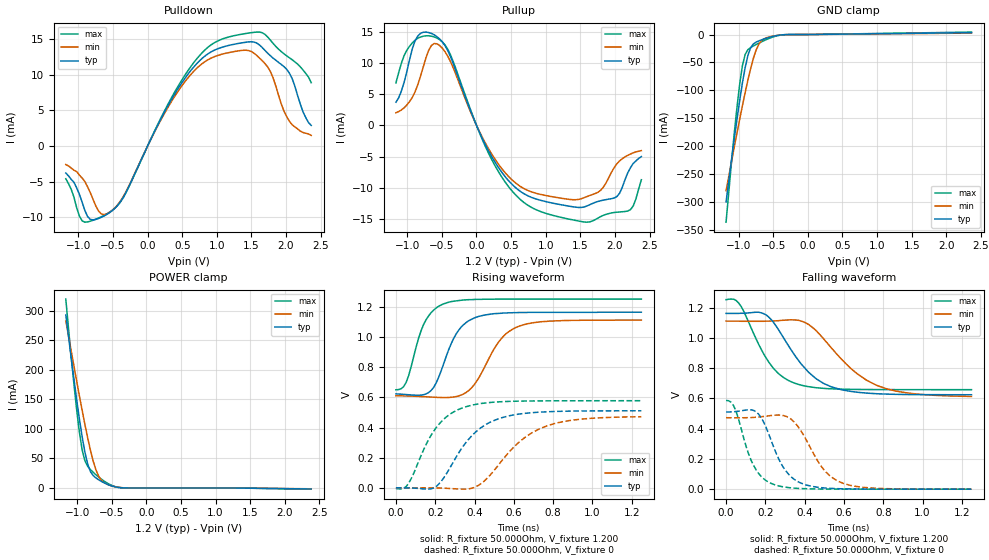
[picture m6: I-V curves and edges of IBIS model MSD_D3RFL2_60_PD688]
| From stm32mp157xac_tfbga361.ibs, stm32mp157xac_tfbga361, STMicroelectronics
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[Model] MSD_D3RFL2_60_PD688
Model_type   I/O
C_comp 2.461pF   2.375pF   2.586pF
Vinh = 820.000mV
Vinl = 380.000mV
Vmeas = 600.000mV
Vref = 600.000mV
[Model Spec]
Vinh   820.000mV   790.000mV   870.000mV
Vinl   380.000mV   350.000mV   430.000mV
Vmeas   600.000mV   570.000mV   650.000mV
Vref   600.000mV   570.000mV   650.000mV
[Temperature Range]   25.000   125.000   -40.000
[Voltage Range]   1.200V   1.140V   1.300V
[GND Clamp Reference]   0.00V   0.00V   0.00V
[Pulldown Reference]   0.00V   0.00V   0.00V
[POWER Clamp Reference]   1.200V   1.140V   1.300V
[Pullup Reference]   1.200V   1.140V   1.300V
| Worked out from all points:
|   slope of the pulldown table from 0 to 0.18 V, typ, clamps not added: 50.1 ohm
|   slope of the pullup table from 0 to 0.18 V, typ, clamps not added: 42.9 ohm
|   GND clamp passes 1 mA (typ) near -0.40 V on its own axis
|   POWER clamp passes 1 mA (typ) near -0.41 V on its own axis
|   rising waveform, R_fixture 50.000Ohm, V_fixture 1.200: 20-80 % time 109ps typ, 140ps min, 91.6ps max; typ from 0.623 V to 1.16 V
|   rising waveform, R_fixture 50.000Ohm, V_fixture 0: 20-80 % time 183ps typ, 224ps min, 153ps max; typ from 0.001 V to 0.511 V
|   falling waveform, R_fixture 50.000Ohm, V_fixture 1.200: 20-80 % time 190ps typ, 242ps min, 153ps max; typ from 1.16 V to 0.625 V
|   falling waveform, R_fixture 50.000Ohm, V_fixture 0: 20-80 % time 113ps typ, 138ps min, 96.4ps max; typ from 0.51 V to 0 V
[GND Clamp]
-1.182V   -299.6mA   -279.7mA   -335.9mA
-1.064V   -187.4mA   -201.8mA   -177.5mA
-984.9mV  -117.9mA   -151.6mA   -88.6mA
-945.5mV  -86.54mA   -127.3mA   -55.77mA
-906.1mV  -59.13mA   -104mA     -35.64mA
-866.7mV  -37.61mA   -81.71mA   -27.22mA
-827.3mV  -23.8mA    -61.15mA   -23.42mA
-748.5mV  -13.62mA   -28.14mA   -17.95mA
-709.1mV  -11.42mA   -17.52mA   -15.44mA
-630.3mV  -7.875mA   -7.542mA   -10.71mA
-472.7mV  -2.454mA   -2.156mA   -3.182mA
2.364V    3.327mA    2.556mA    4.357mA
[Power Clamp]
-1.164V   292.5mA    282.6mA    319.4mA
-1.085V   218.7mA    230.9mA    220.2mA
-1.006V   148.5mA    180.1mA    131.2mA
-966.7mV  115.9mA    155.2mA    93.42mA
-927.3mV  86.16mA    130.9mA    64.04mA
-887.9mV  60.43mA    107.4mA    45.92mA
-809.1mV  27.85mA    64.33mA    31.18mA
-730.3mV  17.06mA    31.16mA    22.45mA
-651.5mV  11.24mA    13.38mA    14.99mA
-533.3mV  4.769mA    4.703mA    6.239mA
-336.4mV  190.8uA    361uA      219.4uA
2.382V    -1.713mA   -1.413mA   -2.032mA
[Pulldown]
-1.182V   -3.8mA     -2.6mA     -4.6mA
-945.5mV  -7.91mA    -4.5mA     -10.52mA
-827.3mV  -10.31mA   -6.57mA    -10.56mA
-669.7mV  -10.02mA   -9.53mA    -9.94mA
-551.5mV  -9.373mA   -9.335mA   -9.299mA
-315.1mV  -6.567mA   -6.465mA   -6.607mA
551.5mV   9.674mA    9.198mA    10.14mA
906.1mV   13.16mA    12.3mA     14.14mA
1.3V      14.39mA    13.35mA    15.61mA
1.733V    13.06mA    11.13mA    15.34mA
2.009V    10.78mA    4.14mA     12.68mA
2.364V    2.9mA      1.5mA      8.9mA
[Pullup]
-1.164V   3.7mA      2.005mA    6.785mA
-1.045V   6.9mA      2.809mA    11.16mA
-887.9mV  13.51mA    5.344mA    13.62mA
-690.9mV  14.84mA    11.99mA    14.32mA
-454.5mV  12.73mA    11.77mA    12.85mA
175.8mV   -4.108mA   -3.772mA   -4.491mA
687.9mV   -10.95mA   -10.12mA   -12.36mA
1.476V    -13.13mA   -11.84mA   -15.3mA
1.791V    -12.06mA   -10.42mA   -14.61mA
1.988V    -11.63mA   -6.784mA   -13.94mA
2.224V    -6.8mA     -4.595mA   -13.49mA
2.382V    -5mA       -4.048mA   -8.7mA
[Ramp]
R_load=50.000Ohm
dV/dt_r   315.030mV/147.500ps  292.319mV/184.000ps  351.210mV/122.500ps
dV/dt_f   315.000mV/152.500ps  292.290mV/192.500ps  351.210mV/124.500ps
[Rising waveform]
R_fixture=50.000Ohm
V_fixture=1.200
V_fixture_min=1.140
V_fixture_max=1.300
0s        622.7mV    610.6mV    650.2mV
52ps      618.5mV    609.3mV    699.2mV
128ps     614.8mV    605.3mV    1.041V
166ps     631.6mV    602.8mV    1.139V
243ps     822.8mV    598.6mV    1.219V
307ps     1.021V     605.2mV    1.239V
370ps     1.107V     644.6mV    1.247V
523ps     1.156V     967.3mV    1.251V
626ps     1.162V     1.071V     1.251V
1.249ns   1.164V     1.112V     1.251V
[Rising waveform]
R_fixture=50.000Ohm
V_fixture=0
0s        574.4uV    127.3uV    -3.509mV
64ps      247.6uV    471.3uV    29.6mV
192ps     -724.5uV   251.1uV    375.7mV
256ps     91.72mV    -2.437mV   469.7mV
345ps     281.3mV    -8.186mV   533.3mV
421ps     386.7mV    17.63mV    556.6mV
485ps     438.8mV    93.5mV     566.6mV
626ps     489.4mV    302.5mV    574.9mV
766ps     504.2mV    409.9mV    576.8mV
1.249ns   510.9mV    471.5mV    577.7mV
[Falling waveform]
R_fixture=50.000Ohm
V_fixture=1.200
V_fixture_min=1.140
V_fixture_max=1.300
0s        1.163V     1.112V     1.254V
77ps      1.164V     1.111V     1.209V
205ps     1.152V     1.112V     865.9mV
268ps     1.053V     1.115V     763.6mV
345ps     894.7mV    1.12V      703.5mV
421ps     772.5mV    1.089V     678.2mV
498ps     698.7mV    992.5mV    666.9mV
638ps     646.4mV    795.6mV    660.4mV
766ps     631.6mV    687.2mV    659.1mV
1.249ns   624.8mV    613.7mV    658.3mV
[Falling waveform]
R_fixture=50.000Ohm
V_fixture=0
0s        510.3mV    472.7mV    587.1mV
39ps      512.5mV    472.4mV    550.9mV
115ps     525.2mV    473.2mV    232.5mV
154ps     510.9mV    476.1mV    125.6mV
243ps     276.1mV    489.2mV    31.31mV
294ps     139.1mV    486.2mV    14.66mV
358ps     55.36mV    427.6mV    5.827mV
498ps     8.363mV    128.7mV    733.7uV
600ps     2.138mV    36.74mV    144uV
1.249ns   -4.24uV    21.19uV    -3.531uV
